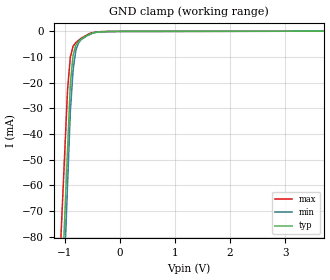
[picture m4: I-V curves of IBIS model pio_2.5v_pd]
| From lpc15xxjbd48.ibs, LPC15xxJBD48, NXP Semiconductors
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[Model] pio_2.5v_pd
Model_type Input
Vinl = 750.000mV
Vinh = 1.75000V
C_comp 598.000fF 598.000fF 598.000fF
| variable typ   min   max
[Voltage Range] 2.50000V 2.25000V 2.75000V
[POWER Clamp Reference] 2.50000V 2.25000V 2.75000V
[GND Clamp Reference] 0.00000V 0.00000V 0.00000V
[Temperature Range]   25   85   -40
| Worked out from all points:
|   GND clamp passes 1 mA (typ) near -0.53 V on its own axis
[GND Clamp]
-2.5V     -841.8mA   -937.4mA   -760.7mA
-950mV    -45.98mA   -59.49mA   -22.46mA
-900mV    -20.31mA   -31.17mA   -9.92mA
-850mV    -9.295mA   -15.13mA   -5.75mA
-800mV    -5.361mA   -7.32mA    -4.325mA
-750mV    -3.856mA   -4.403mA   -3.465mA
-700mV    -2.925mA   -3.175mA   -2.604mA
-550mV    -1.147mA   -1.261mA   -826.7uA
-400mV    -251.9uA   -258.3uA   -178uA
319.2uV   -34.85uA   1.283uA    -12.55uA
5V        123uA      101.1uA    107uA
[POWER Clamp]
-2.5V     0A         0A         0A
5V        0A         0A         0A
